(* Logix 5000 AddOnInstructionDefinition export; software revision 16.04 *)

ADD_ON_INSTRUCTION AMCI_ANG1E_Jog_CCW   (* revision 1.1, vendor AMCI *)
// Revision note:
// Version 1.1 added the slot_axis number and the input parameters can now be tags or discrete values.
VAR_INPUT
   slot_axis_number : INT; {required}
   Programmed_Speed : DINT; {required}
   Acceleration : INT; {required}
   Deceleration : INT; {required}
END_VAR
VAR_OUTPUT
   Jog_CCW_Occurring : BOOL; {required}
END_VAR
VAR_IN_OUT
   AMCI_ANG1E_output_data : INT[10]; {required}
END_VAR
VAR
   Upper_Result_X_1000 : DINT;
   command_data_block : INT[10];
        [0]   // Command Bits MSW
        [1]   // Command Bits LSW
        [2]   // Upper Target Position
        [3]   // Lower Target Position
        [4]   // Upper Programmed Speed
        [5]   // Lower Programmed Speed
   index : INT;
END_VAR

ROUTINE Logic   (* ladder *)
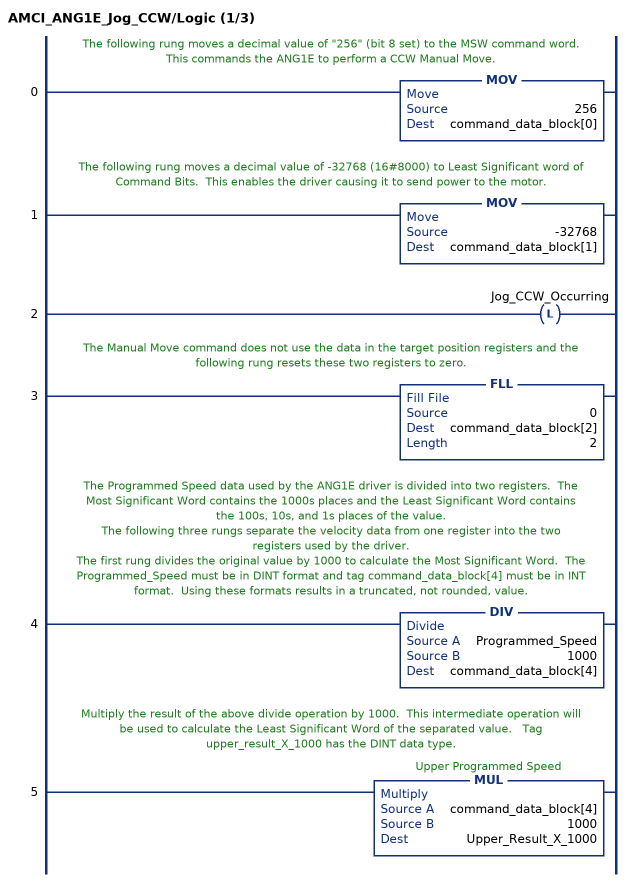
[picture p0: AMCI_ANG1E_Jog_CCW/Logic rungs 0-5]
   // The following rung moves a decimal value of "256" (bit 8 set) to the MSW command word.  This commands the ANG1E to perform a CCW Manual Move.
   0: MOV(256,command_data_block[0]);
   // The following rung moves a decimal value of -32768 (16#8000) to Least Significant word of Command Bits.  This enables the driver causing it to send power to the motor.
   1: MOV(-32768,command_data_block[1]);
   2: OTL(Jog_CCW_Occurring);
   // The Manual Move command does not use the data in the target position registers and the following rung resets these two registers to zero.
   3: FLL(0,command_data_block[2],2);
   // The Programmed Speed data used by the ANG1E driver is divided into two registers.  The Most Significant Word contains the 1000s places and the Least Significant Word contains the 100s, 10s, and 1s places of the value.
   // The following three rungs separate the velocity data from one register into the two registers used by the driver.
   // The first rung divides the original value by 1000 to calculate the Most Significant Word.  The Programmed_Speed must be in DINT format and tag command_data_block[4] must be in INT format.  Using these formats results in a truncated, not rounded, value.
   4: DIV(Programmed_Speed,1000,command_data_block[4]);
   // Multiply the result of the above divide operation by 1000.  This intermediate operation will be used to calculate the Least Significant Word of the separated value.   Tag upper_result_X_1000 has the DINT data type.
   5: MUL(command_data_block[4],1000,Upper_Result_X_1000);
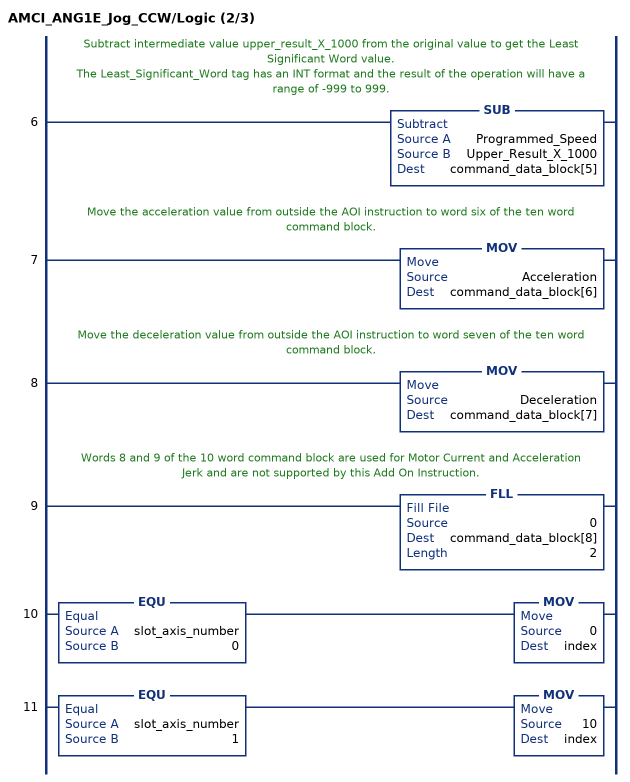
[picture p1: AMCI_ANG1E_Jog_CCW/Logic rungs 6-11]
   // Subtract intermediate value upper_result_X_1000 from the original value to get the Least Significant Word value.
   // The Least_Significant_Word tag has an INT format and the result of the operation will have a range of -999 to 999.
   6: SUB(Programmed_Speed,Upper_Result_X_1000,command_data_block[5]);
   // Move the acceleration value from outside the AOI instruction to word six of the ten word command block.
   7: MOV(Acceleration,command_data_block[6]);
   // Move the deceleration value from outside the AOI instruction to word seven of the ten word command block.
   8: MOV(Deceleration,command_data_block[7]);
   // Words 8 and 9 of the 10 word command block are used for Motor Current and Acceleration Jerk and are not supported by this Add On Instruction.
   9: FLL(0,command_data_block[8],2);
   10: EQU(slot_axis_number,0)MOV(0,index);
   11: EQU(slot_axis_number,1)MOV(10,index);
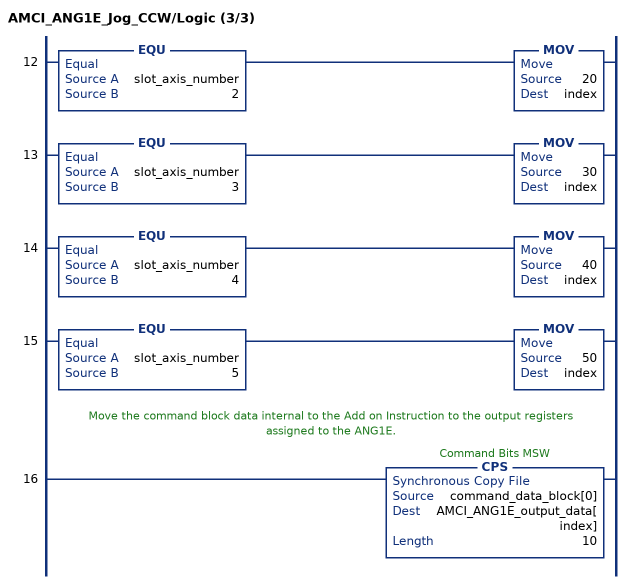
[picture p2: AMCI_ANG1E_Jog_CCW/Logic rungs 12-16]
   12: EQU(slot_axis_number,2)MOV(20,index);
   13: EQU(slot_axis_number,3)MOV(30,index);
   14: EQU(slot_axis_number,4)MOV(40,index);
   15: EQU(slot_axis_number,5)MOV(50,index);
   // Move the command block data internal to the Add on Instruction to the output registers assigned to the ANG1E.
   16: CPS(command_data_block[0],AMCI_ANG1E_output_data[index],10);
END_ROUTINE
END_ADD_ON_INSTRUCTION
